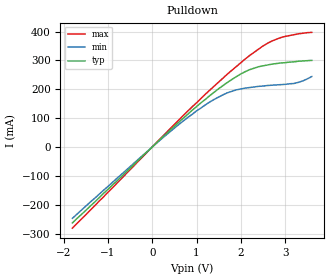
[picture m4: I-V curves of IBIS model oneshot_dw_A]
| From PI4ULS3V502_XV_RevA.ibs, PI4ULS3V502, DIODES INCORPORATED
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[Model]   oneshot_dw_A
Model_type  Open_sink
Vref = 1.8
Rref = 50
Vmeas = 0.9
C_comp   8.966pF   8.863pF   9.079pF
[Voltage Range]   1.80V   1.62V   1.98V
[Temperature Range]   25   85   -40
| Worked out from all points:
|   slope of the pulldown table from 0 to 0.27 V, typ, clamps not added: 6.87 ohm
[Pulldown]
-1.8V     -263mA     -247mA     -281mA
500mV     71.9mA     65.4mA     78mA
1.2V      165mA      146mA      183mA
1.7V      224mA      188mA      253mA
1.9V      244mA      198mA      279mA
2.2V      268mA      206mA      317mA
2.5V      281mA      211mA      350mA
2.7V      287mA      214mA      367mA
2.9V      291mA      216mA      379mA
3.2V      295mA      220mA      389mA
3.4V      298mA      229mA      394mA
3.6V      300mA      244mA      397mA
[Ramp]
| variable   typ   min   max
dV/dt_r   0.95/513.4E-12   0.62/512.7E-12   1.05/512.5E-12
dV/dt_f   0.95/74.3E-12   0.62/96.9E-12   1.05/58.1E-12
R_load = 50
